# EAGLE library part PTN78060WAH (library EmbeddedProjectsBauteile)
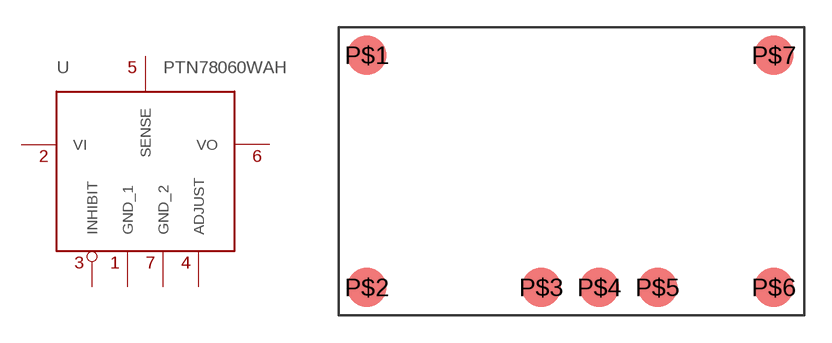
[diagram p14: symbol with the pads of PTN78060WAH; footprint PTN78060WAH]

Designator prefix -

## PTN78060WAH (EP: 400180)  [PTN78060WAH]
P$1  GND_1
P$2  VI
P$3  INHIBIT
P$4  ADJUST
P$5  SENSE
P$6  VO
P$7  GND_2

## Footprint PTN78060WAH (pad centres in mm)
smd 2.16 x 2.16: P$1 -11.175,6.35; P$2 -11.175,-6.35; P$3 -1.65,-6.35; P$4 1.525,-6.35; P$5 4.7,-6.35; P$6 11.05,-6.35; P$7 11.05,6.35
